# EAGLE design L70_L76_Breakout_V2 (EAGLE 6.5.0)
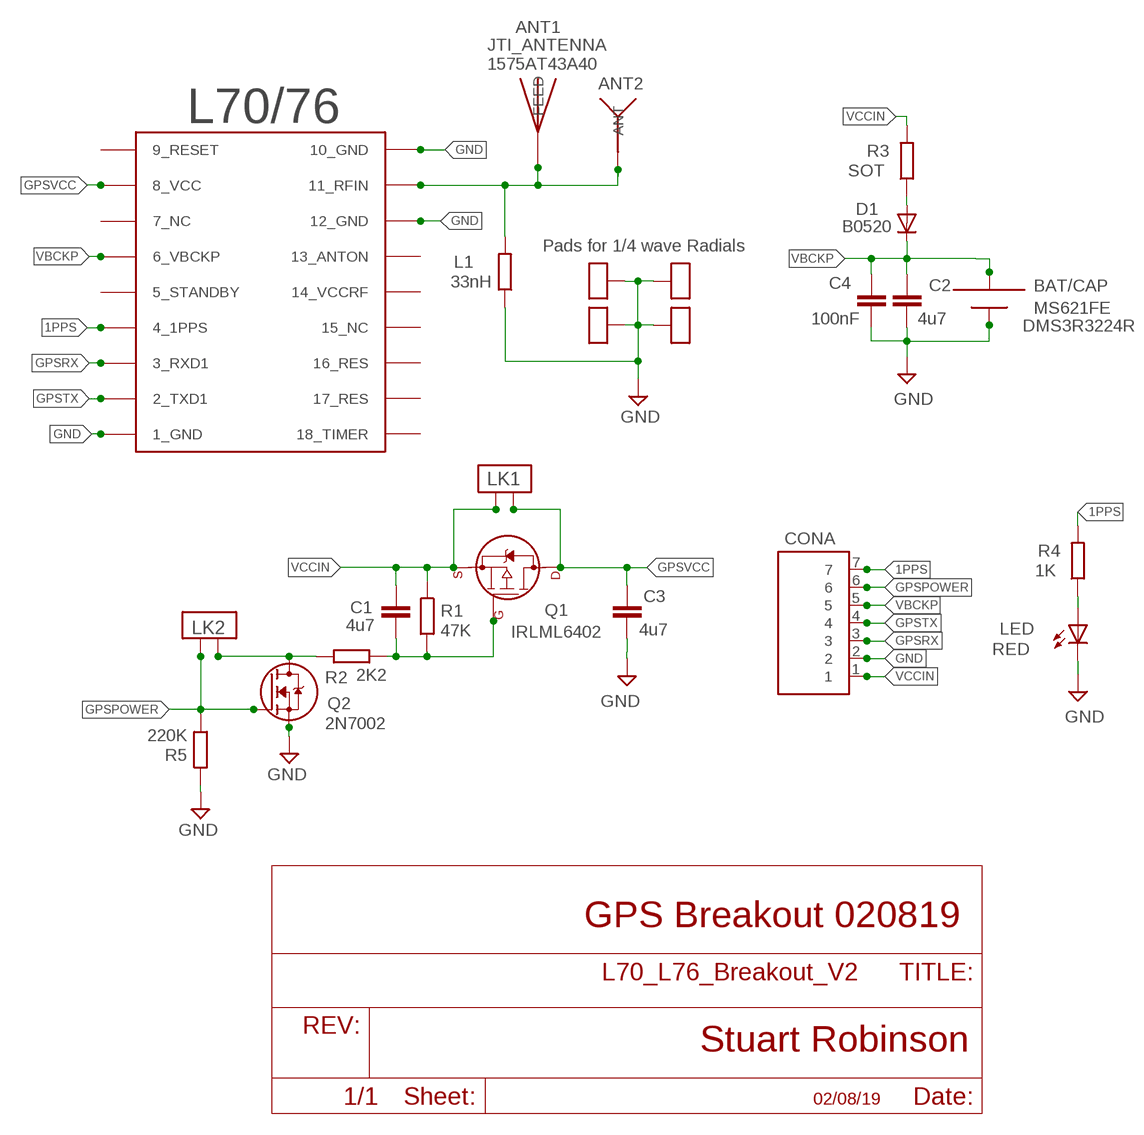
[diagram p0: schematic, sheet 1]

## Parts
ANT1  JTI_ANTENNA-1575AT43A40  [JTI_ANTENNA-1575AT43A40]
ANT2  13MM_CERAMIC_PATCH  [13MM_CERAMIC_PATCH]
BAT/CAP  MS621FE  PCBBATTERY  [PCBBATTERY]
C1  4u7  C805_REDUCED  [C0805_REDUCED]
C2  4u7  C805_REDUCED  [C0805_REDUCED]
C3  4u7  C805_REDUCED  [C0805_REDUCED]
C4  100nF  C805_REDUCED  [C0805_REDUCED]
CONA  7X1  [7X1]
D1  B0520  DIODE-SOD323-R  [SOD323-R]
L1  33nH  R-EU_R0603  [R0603]
L70/76  L70GPS  [L70_GPS]
LED  RED  0805LED  [0805LED]
LK1  PCB_LINK_2  [PCB_LINK2]
LK2  PCB_LINK_2  [PCB_LINK2]
PAD1  ANTPAD2  [ANTPAD2]
PAD2  ANTPAD2  [ANTPAD2]
PAD3  ANTPAD2  [ANTPAD2]
PAD4  ANTPAD2  [ANTPAD2]
Q1  IRLML6402  IRLFL6402  [SOT23@1]
Q2  2N7002  NMOSFET  [SOT23]
R1  47K  R0805_REDUCED  [R0805_REDUCED]
R2  2K2  R0805_REDUCED  [R0805_REDUCED]
R3  SOT  R0805_REDUCED  [R0805_REDUCED]
R4  1K  R0805_REDUCED  [R0805_REDUCED]
R5  220K  R0805_REDUCED  [R0805_REDUCED]

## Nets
1PPS: CONA.7 L70/76.4_1PPS R4.2
GND [GND]: BAT/CAP.-VE C2.2 C3.2 C4.2 CONA.2 L1.1 L70/76.1_GND L70/76.10_GND L70/76.12_GND LED.C PAD1.P$1 PAD2.P$1 PAD3.P$1 PAD4.P$1 Q2.2(S) R5.1
GPSPOWER: CONA.6 LK2.P$1 Q2.1(G) R5.2
GPSRX: CONA.3 L70/76.3_RXD(3_RXD1)
GPSTX: CONA.4 L70/76.2_TXD(2_TXD1)
GPSVCC [gpsdefault]: C3.1 L70/76.8_VCC LK1.P$1 Q1.3(D1)
N$1: C1.2 Q1.1(G1) R1.2 R2.2
N$2: LED.A R4.1
N$4 [gpspower]: D1.A R3.1
N$7: LK2.P$2 Q2.3(D) R2.1
RFIN1 [gpspower]: ANT1.FEED ANT2.P$1(ANT) L1.2 L70/76.11_RFIN
VBCKP [gpspower]: BAT/CAP.+VE C2.1 C4.1 CONA.5 D1.C L70/76.6_VBCKP
VCCIN [GND]: C1.1 CONA.1 LK1.P$2 Q1.2(S1) R1.1 R3.2
Unconnected: L70/76.5_STANDBY L70/76.13_NC(13_ANTON) L70/76.14_VCCRF L70/76.15_NC L70/76.16_RES L70/76.17_RES L70/76.18_NC(18_TIMER)

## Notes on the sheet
- JTI_ANTENNA
  1575AT43A40
- Pads for 1/4 wave Radials
- DMS3R3224R
- GPS Breakout 020819
- 02/08/19

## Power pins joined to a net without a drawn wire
7_NC: L70/76.7_NC
9_RESET: L70/76.9_RESET

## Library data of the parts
ANT1 = Ava2:JTI_ANTENNA-1575AT43A40
ANT2 = LMA2:13MM_CERAMIC_PATCH
BAT/CAP = LMA2:PCBBATTERY
C1-C4 = resistor:C805_REDUCED
CONA = My_Pin_Headers:7X1
D1 = diode:DIODE-: DIODE
L1 = resistor:R-EU_: RESISTOR, European symbol
L70/76 = Ava2:L70GPS
LED = LMA2:0805LED
LK1 LK2 = LMA2:PCB_LINK_2
PAD1-PAD4 = LMA2:ANTPAD2
Q1 = LMA2:IRLFL6402
Q2 = LMA2:NMOSFET
R1-R5 = resistor:R0805_REDUCED

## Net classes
0 default: width 0.152 mm
1 GND: width 0.508 mm
2 gpsdefault: width 0.508 mm
3 gpspower: width 0.508 mm

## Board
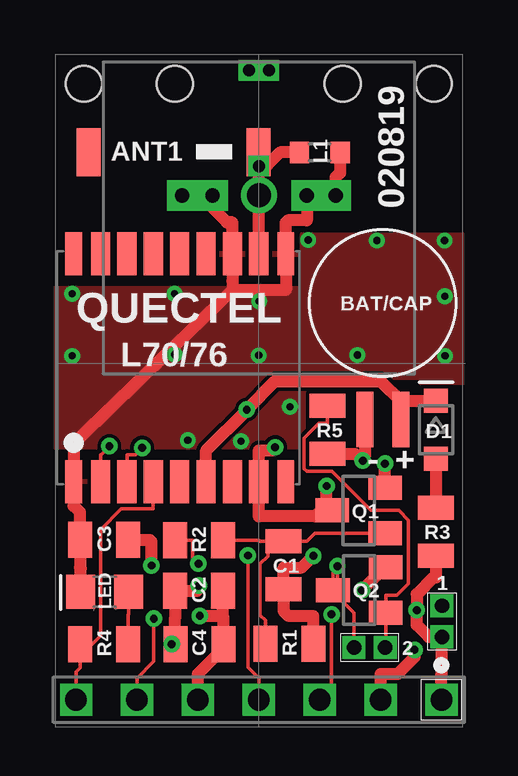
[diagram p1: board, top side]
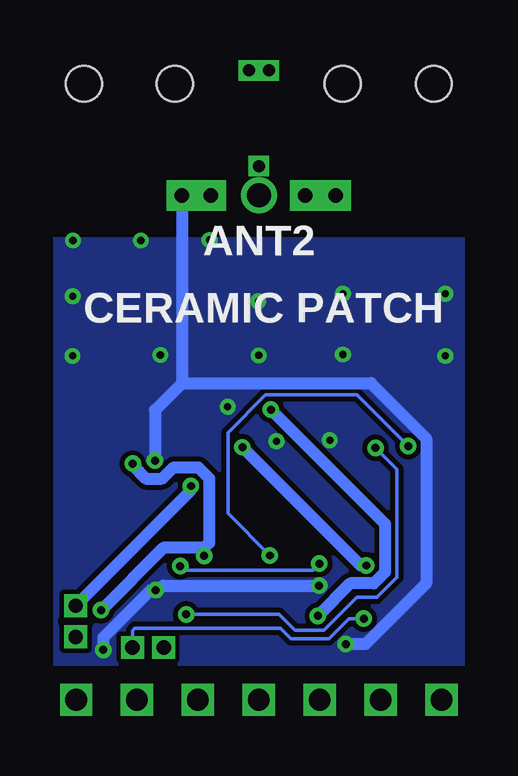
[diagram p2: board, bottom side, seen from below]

No outline drawn. Coordinates in mm, seen from the top.
Copper layers (1*16): Top 0.0356mm / dielectric 1.5011mm / Bottom 0.0356mm
Design rules "LaenPCBOrder *": minimum track width 6mil, minimum drill 13mil, track to track 6mil, track to pad 6mil, pad to pad 6mil, via to via 6mil, smd to smd 6mil, copper to edge 15mil, drill to drill 6mil, minimum pad ring 7mil, minimum via ring 7mil, stop-mask expansion 4mil, vias tented up to drill 1000mil, thermal gap 10mil
Holes 1.5 mm at 1.2,26.8 5,26.8 15.8,26.8 12,26.8
tRestrict: area 0,20.6 to 17,22.3; area 0.4,18.4 to 10.2,18.8; area 0.3,11.1 to 10.2,11.6; area 0,-0.1 to 17.1,2.6; area 0,2.6 to 17.1,10.1; area 0,18.4 to 0.4,18.8; area 0,11.1 to 0.3,11.5; area -0.1,9.9 to 0.5,11.2; area 12.3,11.1 to 15.2,14.4; area 12.1,10.1 to 13.4,11.1; area 10.6,11.7 to 12.4,12.9; area 10.5,12.4 to 10.6,12.8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
bRestrict: area 0,0.2 to 17,2.4; area 0,20.6 to 16.9,22.2

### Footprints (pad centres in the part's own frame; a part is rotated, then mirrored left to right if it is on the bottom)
JTI_ANTENNA-1575AT43A40 = smd 1 x 2: FEED -3.175,0; NC 3.925,0
13MM_CERAMIC_PATCH = drill 1: P$1 0,0.95
PCBBATTERY = smd 2.3 x 0.7: +VE 4.85,0.75; -VE 4.85,-0.75
C0805_REDUCED = smd 1 x 1.5: 1 -1,0; 2 1,0
7X1 = drill 0.9 square: 1 -7.62,0; 2 -5.08,0; 3 -2.54,0; 4 0,0; 5 2.54,0; 6 5.08,0; 7 7.62,0
SOD323-R = smd 1 x 1: A 1.2,0; C -1.2,0
R0603 = smd 0.8 x 0.9: 1 -0.85,0; 2 0.85,0
L70_GPS = smd 1.8 x 0.7: 1_GND 4.95,-4.475; 9_RESET 4.95,4.375; 10_GND -4.55,4.375; 18_NC -4.55,-4.475 | smd 1.8 x 0.8: 2_TXD 4.95,-3.35; 3_RXD 4.95,-2.25; 4_1PPS 4.95,-1.15; 5_STANDBY 4.95,-0.05; 6_VBCKP 4.95,1.05; 7_NC 4.95,2.15; 8_VCC 4.95,3.25; 11_RFIN -4.55,3.25; 12_GND -4.55,2.15; 13_NC -4.55,1.05; 14_VCCRF -4.55,-0.05; 15_NC -4.55,-1.15; 16_RES -4.55,-2.25; 17_RES -4.55,-3.35
0805LED = smd 1.4 x 1.2: A 0,-1; C 0,1
PCB_LINK2 = drill 0.6 square: P$1 -0.65,0; P$2 0.65,0
ANTPAD2 = drill 0.6 pad 1.27 square: P$1 0,0
SOT23@1 = smd 1 x 1.4: 1 -0.95,-1.1; 2 0.95,-1.1; 3 0,1.1
SOT23 = smd 1 x 1.4: 1 -0.95,-1.1; 2 0.95,-1.1; 3 0,1.1
R0805_REDUCED = smd 1 x 1.5: 1 -1,0; 2 1,0

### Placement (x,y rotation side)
ANT1  5.32,23.94 180 top
ANT2  8.5,21.21 0 top
BAT/CAP  13.67,17.66 270 top
C1  9.53,6.73 90 top
C2  6,5.67 180 top
C3  2.04,7.79 180 top
C4  6.02,3.45 180 top
CONA  8.5,1.13 180 top
D1  15.89,12.38 270 top
L1  11.04,23.94 180 top
L70/76  5.25,15.17 270 top
LED  2.07,5.63 90 top
LK1  16.14,4.4 270 top
LK2  13.12,3.31 180 top
PAD1  5.3,22.15 0 top
PAD2  6.57,22.15 0 top
PAD3  10.5,22.15 0 top
PAD4  11.71,22.15 0 top
Q1  12.66,9.02 90 top
Q2  12.69,5.7 90 top
R1  9.77,3.46 180 top
R2  6,7.78 0 top
R3  15.89,8.14 270 top
R4  2.05,3.44 180 top
R5  11.37,12.38 90 top

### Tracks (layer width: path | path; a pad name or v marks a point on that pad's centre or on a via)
1PPS
  Top 0.152: 1.05,2.95 1.9,3.8 1.9,8.22 2.77,9.09 4.1,9.09 L70/76.4_1PPS | 1.05,2.95 1.05,2.46 0.88,2.29 CONA.7 | R4.2 1.05,2.95
GND  (via drill 0.3, 0.33 pad 0.69)
  Top 0.508: 7.4,18.2 0.78,11.79 L70/76.1_GND 0.78,9.21 1.04,8.95 C3.2 1.04,6.63 1.07,6.6 LED.C | 7.4,18.2 7.4,18.58 L70/76.12_GND 7.4,21.03 7.17,21.03 6.57,21.63 | 7.4,18.2 9.62,18.2 L70/76.10_GND 9.62,20.37 9.62,21.03 9.71,21.11 10.5,21.11 PAD3.P$1 11.54,22.15 PAD4.P$1 11.71,22.9 11.89,23.08 L1.1 | PAD1.P$1 6.34,22.15 6.34,21.86 6.57,21.63 | PAD2.P$1 6.57,21.63 | v14.99,3.21 14.99,2.91 14.29,2.21 13.58,2.21 CONA.2 | 5,3.45 v4.87,3.45 | C4.2 5,3.45 | 5,3.45 5,4.51 C2.2 5.91,5.67 5.91,5.81 v5.99,5.89 | BAT/CAP.-VE 12.92,11.25 12.84,11.25 | R5.1 12.53,11.38 12.65,11.25 12.84,11.25 | v12.8,5.7 13.7,6.6 Q2.2 | v12.84,11.09 12.84,11.25
  Bottom 0.508: 11.71,14.32 3.82,14.32 1.52,12.01 1.52,5.99 4.05,3.45 v4.87,3.45 | v14.99,3.21 14.99,3.72 13.01,5.7 v12.8,5.7 12.48,5.89 v5.99,5.89 | 11.71,14.32 12.84,13.2 v12.84,11.09 | PAD4.P$1 11.71,14.32
  other vias: 16.25,20.27 10.56,20.29 16.27,15.46 0.72,15.46 8.5,15.48 4.99,15.52 12.61,15.5 13.42,20.27 16.26,17.94 0.72,18.05 4.99,18.05 8.52,17.74 5.54,11.94 9.8,13.34 7.76,11.9
  pour Bottom (isolate 0.2): 0,21.99 17,21.99 17,0 0,0
  pour Top: 0,22.07 17,22.07 17,0 0,0
GPSPOWER  (via drill 0.33 pad 0.69)
  Top 0.152: R5.2 11.37,12.65 11.01,12.65 10.39,12.04 10.39,10.77 10.51,10.65 11.55,10.65 13.18,9.02 14.33,9.02 14.74,8.62 14.74,5.97 14.25,5.48 13.79,5.48 Q2.1 13.79,3.33 LK2.P$1 | CONA.6 3.42,2.03 4.12,2.73 v4.12,4.51
  Bottom 0.152: LK2.P$1 13.77,4.02 13.68,4.11 7.59,4.11 7.15,3.67 5.58,3.67 4.75,4.51 v4.12,4.51
GPSRX  (via drill 0.33 pad 0.69)
  Top 0.152: L70/76.3_RXD 3,11.35 3.35,11.35 v3.64,11.63 | v11.53,4.69 11.53,1.62 CONA.3
  Bottom 0.152: v3.64,11.63 2.74,10.73 2.74,6.24 3.58,5.4 4.41,5.4 5.79,4.03 7,4.03 7.66,4.69 v11.53,4.69
GPSTX  (via drill 0.33 pad 0.69)
  Top 0.152: v8.04,7.14 8.04,2.49 8.5,2.03 CONA.4 | L70/76.2_TXD 1.9,11.35 1.92,11.35 v2.27,11.7
  Bottom 0.152: v2.27,11.7 4.41,13.84 8.21,13.84 9.79,12.26 9.79,8.89 v8.04,7.14
GPSVCC  (via drill 0.33 pad 0.69)
  Top 0.508: v9.18,11.65 9.06,11.53 8.5,11.53 L70/76.8_VCC 8.5,8.77 10.85,8.77 10.99,8.91 11.22,8.91 11.33,9.02 | Q1.3 11.33,9.02 | 11.33,9.02 v11.33,10.04 | C3.1 3.95,7.79 4.02,7.72 v4.02,6.73
  Bottom 0.508: v4.02,6.73 4.26,6.73 v9.18,11.65 | LK1.P$1 11.33,9.86 v11.33,10.04 | v11.33,10.04
N$1
  Top 0.152: R1.2 8.77,4.44 8.55,4.66 8.55,6.8 8.87,7.12 8.87,7.73 | 8.87,7.73 8.55,7.73 8.5,7.78 R2.2 | 8.87,7.73 C1.2 10.51,7.73 10.85,8.07 Q1.1
N$2
  Top 0.152: LED.A 3.07,4.7 3.05,4.68 R4.1
N$3  (via drill 0.5)
  other vias: 8.08,27.36
N$4
  Top 0.508: D1.A R3.1
N$5  (via drill 0.5)
  other vias: 8.92,27.36
N$6  (via drill 0.5)
  other vias: 8.5,23.37
N$7  (via drill 0.33 pad 0.69)
  Top 0.152: Q2.3 11.59,6.43 11.78,6.43 | R2.1 5.73,7.78 5.73,7.05 v5.98,6.8 | 11.78,6.43 11.78,5.45 12.47,4.76 LK2.P$2 | v11.78,6.7 11.78,6.43
  Bottom 0.152: v5.98,6.8 6.25,6.53 11.61,6.53 v11.78,6.7
RFIN1
  Top 0.508: L1.2 9.38,23.94 8.84,23.4 8.49,23.4 | 8.49,23.4 8.49,22.53 8.5,22.53 ANT2.P$1 L70/76.11_RFIN | ANT1.FEED 8.49,23.4
VBCKP  (via drill 0.33 pad 0.69)
  Top 0.508: CONA.5 5.96,2.21 7,3.25 7,3.45 | 7,4.63 7,3.45 | C4.1 7,3.45 | v6.04,4.63 7,4.63 | 7,4.63 C2.1 | 14.42,13.59 13.6,14.41 9.18,14.41 v8,13.22 6.3,11.53 L70/76.6_VBCKP | BAT/CAP.+VE 14.42,13.59 | 14.42,13.59 14.97,13.59 14.98,13.58 D1.C
  Bottom 0.508: v8,13.22 3.24,8.46 3.24,6.45 3.71,5.98 4.69,5.98 v6.04,4.63
VCCIN  (via drill 0.33 pad 0.69)
  Top 0.508: 16.12,3.75 15.58,3.75 15.08,4.25 v15.08,4.87 15.08,5.53 15.79,6.23 15.89,6.23 R3.2 | LK1.P$2 16.12,3.75 | 16.12,3.75 16.12,2.21 CONA.1 | R1.1 10.77,4.62 9.74,4.62 9.53,4.82 C1.1 9.53,6.64 10.29,6.64 v10.78,7.13 | Q1.2 v13.76,10.97
  Bottom 0.508: 10.78,7.46 12.49,7.46 v15.08,4.87 | v13.76,10.97 13.76,10.89 13.21,10.35 12.53,10.35 12.05,10.82 11.03,10.82 10.57,10.36 10.57,7.67 10.78,7.46 | v10.78,7.13 10.78,7.46

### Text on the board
tNames: ANT1 | L1 | 020819 | QUECTEL | BAT/CAP | L70/76 | R5 | D1 | - | + | Q1 | R3 | C3 | R2 | C1 | Q2 | 1 | LED | C2 | 2 | R4 | C4 | R1
bNames: ANT2 | CERAMIC PATCH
